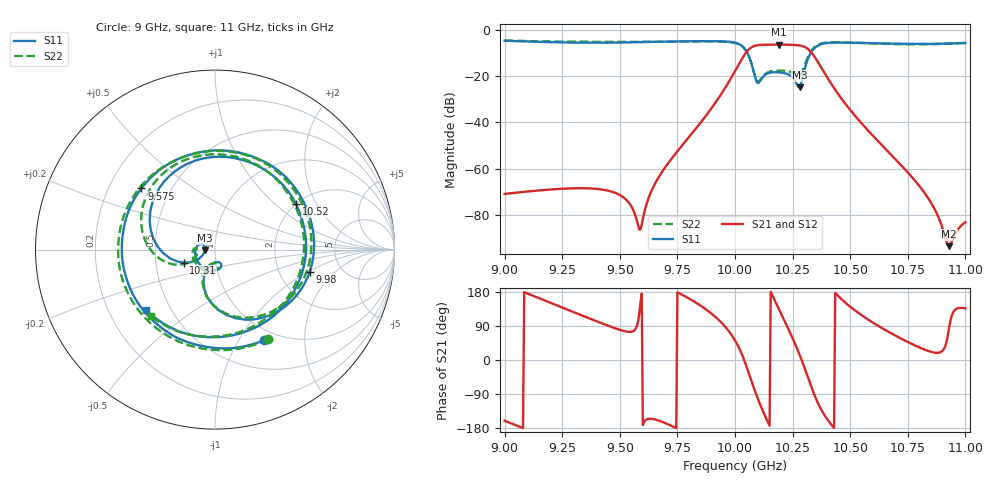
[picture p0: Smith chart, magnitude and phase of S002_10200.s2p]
# Hz S DB R 50
! Planar, S50180, , 20.4.1/1
! Date: 14.11.2021 15:37:17
! Data: Format (Calibration Info)
! Freq	S11:dB/Ang(--)	S21:dB/Ang(--)	S12:dB/Ang(--)	S22:dB/Ang(--)
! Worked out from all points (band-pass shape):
!   401 points, 9 GHz to 11 GHz, reference 50 ohm
!   highest |S21| = -6.48 dB at 10.19 GHz (marker M1); lowest = -93.5 dB at 10.93 GHz (marker M2)
!   |S21| within 3 dB of the highest: 10.05 GHz to 10.33 GHz (275.7 MHz wide, 2.71 % of centre)
!   lowest |S11| = -24.9 dB at 10.28 GHz (marker M3), VSWR 1.12, Z = 44.7 - j0.259 ohm
!   |S11| at or under -10 dB: 10.05 GHz to 10.33 GHz (276.6 MHz wide, 2.71 % of centre)
!   |S22| runs from -22.5 to -4.7 dB; largest |S21 - S12| = 0.00058
!   S11 on the Smith chart (normalised r, x): 9 GHz: 0.85, -1.29; 9.575 GHz: 0.34, +0.32; 9.98 GHz: 2.97, -1.03; 10.31 GHz: 0.70, -0.10; 10.52 GHz: 2.01, +1.38; 11 GHz: 0.36, -0.33
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9e9  -4.82 -61.9  -70.94 -160.3  -70.95 -160.3  -4.72 -59.4
9.335e9  -5.67 -152.6  -68.48 117.7  -68.48 117.7  -5.31 -146.8
9.49e9  -5.63 164.3  -70.91 81.5  -70.92 81.5  -5.35 172.0
9.575e9  -5.46 140.3  -82.86 90.8  -82.87 90.8  -5.32 149.1
9.67e9  -5.27 112.8  -63.53 -160.1  -63.53 -160.1  -5.29 122.7
9.85e9  -4.98 53.4  -40.26 143.7  -40.27 143.7  -5.09 63.3
9.98e9  -5.32 -13.1  -21.43 70.5  -21.44 70.5  -5.51 -7.9
1e10  -5.66 -29.5  -17.95 51.8  -17.95 51.8  -5.84 -25.6
1.0055e10  -10.38 -93.2  -9.11 -26.1  -9.11 -26.1  -10.45 -93.6
1.01e10  -23.13 -82.8  -6.75 -103.6  -6.76 -103.6  -22.53 -91.7
1.0145e10  -18.79 -85.6  -6.52 -167.0  -6.53 -167.0  -18.41 -98.4
1.019e10  -18.48 -133.7  -6.48 135.2  -6.48 135.2  -17.69 -139.8
1.0235e10  -19.52 175.1  -6.57 77.4  -6.57 77.4  -18.07 -175.0
1.028e10  -24.95 -177.1  -6.88 14.6  -6.88 14.5  -20.10 -170.7
1.031e10  -14.46 -157.5  -7.94 -34.5  -7.95 -34.5  -13.36 -156.8
1.0335e10  -9.18 170.2  -10.35 -77.0  -10.36 -77.0  -8.65 178.1
1.0405e10  -5.78 94.3  -21.44 -160.3  -21.44 -160.3  -5.57 108.5
1.052e10  -5.72 29.2  -37.12 131.2  -37.13 131.2  -5.74 43.6
1.067e10  -6.07 -30.1  -53.26 73.0  -53.26 73.0  -6.23 -19.2
1.088e10  -6.16 -102.2  -80.30 19.0  -80.31 19.0  -6.25 -96.1
1.093e10  -6.04 -117.8  -93.50 87.2  -93.51 87.1  -6.05 -112.2
1.1e10  -5.83 -139.0  -83.17 136.2  -83.17 136.1  -5.76 -133.9
